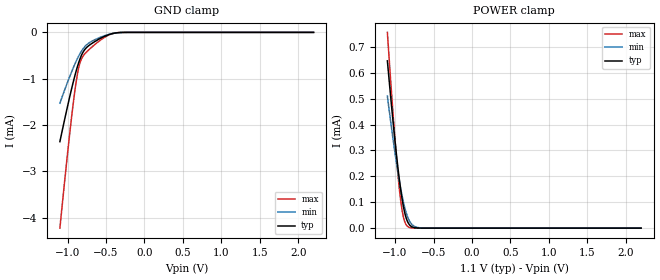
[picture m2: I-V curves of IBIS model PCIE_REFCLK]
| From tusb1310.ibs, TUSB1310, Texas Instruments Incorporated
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|   PCIE_REFCLK Input model
[Model]   PCIE_REFCLK
Model_type   Input
Vinl = 0.35V
Vinh = 0.715V
|   typ   min   max
|   (nom PVT)   (Fast PVT)   (slow PVT)
C_comp   73.45fF   52.85fF   80.72fF
[Voltage Range]   1.1   0.99   1.155
[Temperature Range]   27   105   -40
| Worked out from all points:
|   GND clamp passes 1 mA (typ) near -0.92 V on its own axis
[GND Clamp]
|   Voltage   I(typ)   I(min)   I(max)
-1.1V     -2.359mA   -1.529mA   -4.225mA
-1.017V   -1.723mA   -1.15mA    -2.883mA
-951.1mV  -1.242mA   -866.4uA   -1.877mA
-901.5mV  -913.9uA   -671.3uA   -1.218mA
-860.2mV  -677.2uA   -526.5uA   -803.7uA
-827.1mV  -525.2uA   -426.9uA   -604.5uA
-794mV    -414.7uA   -345.3uA   -500.3uA
-727.8mV  -291.4uA   -236.6uA   -383.1uA
-603.8mV  -157.8uA   -127.1uA   -206.5uA
-454.9mV  -44.45uA   -40.66uA   -51.16uA
-322.6mV  -4.162uA   -5.754uA   -2.74uA
2.2V      0A         0A         0A
[POWER Clamp]
|   Voltage   I(typ)   I(min)   I(max)
-1.1V     645.7uA    509.6uA    755.7uA
-1.05V    485.7uA    396.3uA    539.8uA
-1.009V   360.3uA    307.1uA    372.1uA
-975.9mV  267.5uA    240.6uA    250.8uA
-942.9mV  184.4uA    179.7uA    147.7uA
-918mV    130.7uA    138.7uA    87.4uA
-893.2mV  86.2uA     102.8uA    45.19uA
-868.4mV  52.4uA     72.55uA    20.51uA
-835.3mV  23.78uA    42.03uA    6.222uA
-760.9mV  2.883uA    9.128uA    349.8nA
-645.1mV  86.5nA     597.6nA    3.785nA
2.2V      0A         0A         0A
